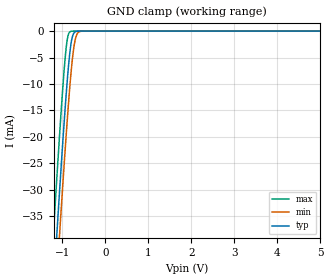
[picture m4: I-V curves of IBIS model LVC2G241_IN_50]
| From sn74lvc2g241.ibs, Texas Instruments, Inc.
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[Model]   LVC2G241_IN_50
Model_type  Input
Vinl=1.35
Vinh=3.85
| variable   typ   min   max
C_comp   3.21pF   2.51pF   4.35pF
[Temperature Range]   40   100   -40
| Ambient temperature   25   85   -40
[Voltage range]   5   4.5   5.5
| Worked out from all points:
|   GND clamp passes 1 mA (typ) near -0.77 V on its own axis
[GND Clamp]
| LVC2G241D_IN_50
|   Voltage   I(typ)   I(min)   I(max)
-5V       -583.8mA   -590.8mA   -575.1mA
-1.21V    -48.93mA   -57.22mA   -38.3mA
-1.13V    -38.42mA   -46.71mA   -27.77mA
-1.07V    -30.71mA   -38.96mA   -20.13mA
-1.05V    -28.19mA   -36.42mA   -17.65mA
-915mV    -12.21mA   -19.95mA   -3.333mA
-870mV    -7.651mA   -14.9mA    -891.1uA
-815mV    -3.252mA   -9.299mA   -87.06uA
-770mV    -1.128mA   -5.445mA   -10.73uA
-705mV    -146.7uA   -1.723mA   -505nA
-575mV    -1.597uA   -52.97uA   -1.117nA
5V        9.69pA     12.83pA    9.218pA
